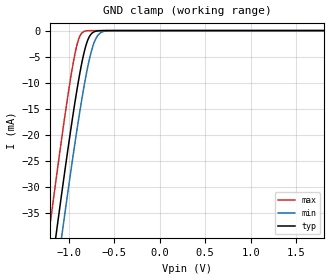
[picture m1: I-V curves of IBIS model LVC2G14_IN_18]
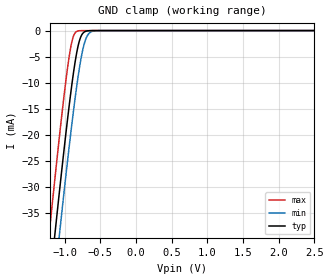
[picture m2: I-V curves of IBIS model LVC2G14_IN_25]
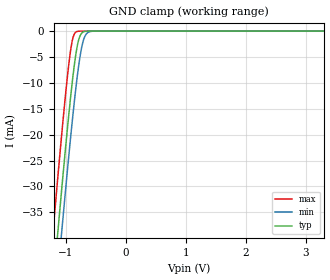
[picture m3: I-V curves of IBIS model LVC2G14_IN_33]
| TEXAS INSTRUMENTS INCORPORATED
| Standard Linear and Logic Group
| IBIS Model of SN74LVC2G14
| DUAL SCHMITT-TRIGGER INVERTER
| This file contains package information for the following:
|  SOT 6-pin (DCK) package as [Component] LVC2G14_DCK
|  SOT 6-pin (DBV) package as [Component] LVC2G14_DBV
|  NanoStar WCSP 6-pin (YEA) package as [Component] LVC2G14_YEA
|  NanoFree WCSP 6-pin (YZA) package as [Component] LVC2G14_YZA
|  NanoStar WCSP 6-pin (YEP) package as [Component] LVC2G14_YEP
|  NanoFree WCSP 6-pin (YZP) package as [Component] LVC2G14_YZP
| This device can be powered at the following Vccs:
|  1.8 volt Vcc
|  2.5 volt Vcc
|  3.3 volt Vcc
|  5 volt Vcc
| This file provides unique models under the [Model Selector] for each Vcc.
| For operation at a specific Vcc, select the appropriate model after each
| [Model Selector] keyword.
[IBIS Ver]   3.2
[Comment char]  |_char
[File Name]   sn74lvc2g14.ibs
[File Rev]   1.2 | d_die
[Date]   August 18, 2003
[Source]   Data created from TI-SPICE simulations at TI-SLL.
[Notes]   The following is an IBIS list for the LVC2G14.
   Please contact sllibis@ti.com with questions and
   comments concerning SLL IBIS models.
   -Due to the fact that the device is 5-V input/output
   tolerant, the output model has some non-monotonic
   warnings.
   -Power clamp data deleted as there is no power-clamp diode.
[Disclaimer] Property of Texas Instruments Incorporated.  Unauthorized
   reproduction and/or distribution is strictly prohibited.
   This product is protected under copyright law.
   Created  2002, (C) Copyright  2002, Texas Instruments
   Incorporated, All Rights Reserved
   UNLESS THERE IS A SIGNED, WRITTEN AGREEMENT TO THE
   CONTRARY, TEXAS INSTRUMENTS (TI) IS PROVIDING THE IBIS
   MODELS  AND WITHOUT ANY WARRANTY, EXPRESSED OR
   IMPLIED.  TI assumes no liability for:
   1) the accuracy of the IBIS models provided to your
   company;
   2) the proper functioning of these IBIS Models in your
   design or for any resulting applications; or
   3) infringement of patents, copyrights or intellectual
   property rights resulting from your use of these IBIS
   models.
   TI provides IBIS Models as a service to our customers.
   You and your company shall not distribute, sell or give
   these models to anyone else without prior written
   permission from TI.
   TI reserves the right to make changes to our products or
   to discontinue any semiconductor product or service
   without notice, and advises our customers to obtain the
   latest version of relevant information to verify, before
   placing orders, that the information being relied on is
   current.
   Please be aware that your receipt and use of the IBIS
   information provided shall serve as acceptance of these
   terms and conditions.  If you do not accept these terms,
   you should return or destroy the IBIS models and any
   other accompanying information immediately.
| Component LVC2G14_DCK 6-pin SOT
[Component]   LVC2G14_DCK
[Manufacturer]   Texas Instruments, Inc.
[Package]
|   typ   min   max
R_pkg   1.400e-02   1.100e-02   2.100e-02
L_pkg   9.480e-10   7.840e-10   1.103e-09
C_pkg   1.910e-13   1.670e-13   2.050e-13
[Pin]   signal_name   model_name   R_pin   L_pin   C_pin
1   1A   LVC2G14_IN   1.300e-02   9.840e-10   1.960e-13
2   GND   GND   2.100e-02   1.103e-09   2.050e-13
3   2A   LVC2G14_IN   1.100e-02   9.980e-10   1.970e-13
4   2Y   LVC2G14_OUT   1.300e-02   9.040e-10   1.900e-13
5   VCC   POWER   1.500e-02   7.840e-10   1.670e-13
6   1Y   LVC2G14_OUT   1.200e-02   9.160e-10   1.950e-13
| Component LVC2G14_DBV 6-pin SOT
[Component]   LVC2G14_DBV
[Manufacturer]   Texas Instruments, Inc.
[Package]
|   typ   min   max
R_pkg   2.500e-02   1.900e-02   3.700e-02
L_pkg   1.524e-09   1.260e-09   1.751e-09
C_pkg   2.450e-13   1.980e-13   2.640e-13
[Pin]   signal_name   model_name   R_pin   L_pin   C_pin
1   1A   LVC2G14_IN   2.100e-02   1.405e-09   2.460e-13
2   GND   GND   3.700e-02   1.751e-09   2.630e-13
3   2A   LVC2G14_IN   2.600e-02   1.493e-09   2.470e-13
4   2Y   LVC2G14_OUT   1.900e-02   1.620e-09   2.640e-13
5   VCC   POWER   2.400e-02   1.260e-09   1.980e-13
6   1Y   LVC2G14_OUT   2.100e-02   1.617e-09   2.500e-13
| Component LVC2G14_YEA 6-pin NanoStar WCSP
[Component]   LVC2G14_YEA
[Manufacturer]   Texas Instruments, Inc.
[Package]
|   typ   min   max
R_pkg   0.001   0.001   0.001
L_pkg   1.021nH   1.021nH   1.021nH
C_pkg   0.047pF   0.046pF   0.047pF
[Pin]   signal_name   model_name   R_pin   L_pin   C_pin
1   1A   LVC2G14_IN   0.001   0.021nH   0.046pF
2   GND   GND   0.001   0.021nH   0.047pF
3   2A   LVC2G14_IN   0.001   0.021nH   0.046pF
4   2Y   LVC2G14_OUT   0.001   0.021nH   0.046pF
5   VCC   POWER   0.001   0.021nH   0.047pF
6   1Y   LVC2G14_OUT   0.001   0.021nH   0.046pF
| Component LVC2G14_YZA 6-pin NanoFree WCSP
[Component]   LVC2G14_YZA
[Manufacturer]   Texas Instruments, Inc.
[Package]
|   typ   min   max
R_pkg   0.001   0.001   0.001
L_pkg   1.021nH   1.021nH   1.021nH
C_pkg   0.047pF   0.046pF   0.047pF
[Pin]   signal_name   model_name   R_pin   L_pin   C_pin
1   1A   LVC2G14_IN   0.001   0.021nH   0.046pF
2   GND   GND   0.001   0.021nH   0.047pF
3   2A   LVC2G14_IN   0.001   0.021nH   0.046pF
4   2Y   LVC2G14_OUT   0.001   0.021nH   0.046pF
5   VCC   POWER   0.001   0.021nH   0.047pF
6   1Y   LVC2G14_OUT   0.001   0.021nH   0.046pF
| Component LVC2G14_YEP 6-pin NanoStar WCSP
[Component]   LVC2G14_YEP
[Manufacturer]   Texas Instruments, Inc.
[Package]
|   typ   min   max
R_pkg   0.001   0.001   0.001
L_pkg   1.021nH   1.021nH   1.021nH
C_pkg   0.047pF   0.046pF   0.047pF
[Pin]   signal_name   model_name   R_pin   L_pin   C_pin
1   1A   LVC2G14_IN   0.001   0.021nH   0.046pF
2   GND   GND   0.001   0.021nH   0.047pF
3   2A   LVC2G14_IN   0.001   0.021nH   0.046pF
4   2Y   LVC2G14_OUT   0.001   0.021nH   0.046pF
5   VCC   POWER   0.001   0.021nH   0.047pF
6   1Y   LVC2G14_OUT   0.001   0.021nH   0.046pF
| Component LVC2G14_YZP 6-pin NanoFree WCSP
[Component]   LVC2G14_YZP
[Manufacturer]   Texas Instruments, Inc.
[Package]
|   typ   min   max
R_pkg   0.001   0.001   0.001
L_pkg   1.021nH   1.021nH   1.021nH
C_pkg   0.047pF   0.046pF   0.047pF
[Pin]   signal_name   model_name   R_pin   L_pin   C_pin
1   1A   LVC2G14_IN   0.001   0.021nH   0.046pF
2   GND   GND   0.001   0.021nH   0.047pF
3   2A   LVC2G14_IN   0.001   0.021nH   0.046pF
4   2Y   LVC2G14_OUT   0.001   0.021nH   0.046pF
5   VCC   POWER   0.001   0.021nH   0.047pF
6   1Y   LVC2G14_OUT   0.001   0.021nH   0.046pF
| Model LVC2G14_IN
[Model Selector]   LVC2G14_IN
LVC2G14_IN_18   1.8 volt Vcc
LVC2G14_IN_25   2.5 volt Vcc
LVC2G14_IN_33   3.3 volt Vcc
LVC2G14_IN_50   5 volt Vcc
| Model LVC2G14_OUT
[Model Selector]   LVC2G14_OUT
LVC2G14_OUT_18   1.8 volt Vcc
LVC2G14_OUT_25   2.5 volt Vcc
LVC2G14_OUT_33   3.3 volt Vcc
LVC2G14_OUT_50   5 volt Vcc
| Models and submodels in the file (8): LVC2G14_IN_18 (Input), LVC2G14_IN_25 (Input), LVC2G14_IN_33 (Input), LVC2G14_IN_50 (Input), LVC2G14_OUT_18 (Output), LVC2G14_OUT_25 (Output), LVC2G14_OUT_33 (Output), LVC2G14_OUT_50 (Output)
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[Model]   LVC2G14_IN_18
Model_type  Input
Vinl=0.7
Vinh=1.4
| variable   typ   min   max
C_comp   3.94pF   3.19pF   4.85pF
[Temperature Range]   40   100   -40
| Ambient temperature   25   85   -40
[Voltage range]   1.8   1.65   1.95
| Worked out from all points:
|   GND clamp passes 1 mA (typ) near -0.77 V on its own axis
[GND Clamp]
| LVC2G14_IN_18
|   Voltage   I(typ)   I(min)   I(max)
-5.5V     -655.2mA   -662.2mA   -646.6mA
-1.215V   -49.6mA    -57.88mA   -38.96mA
-1.135V   -39.07mA   -47.36mA   -28.42mA
-1.075V   -31.35mA   -39.6mA    -20.75mA
-1.055V   -28.82mA   -37.05mA   -18.27mA
-955mV    -16.68mA   -24.66mA   -6.874mA
-885mV    -9.098mA   -16.55mA   -1.486mA
-825mV    -3.922mA   -10.26mA   -137.1uA
-780mV    -1.472mA   -6.227mA   -17.15uA
-715mV    -205.4uA   -2.128mA   -808.5nA
-650mV    -22.01uA   -443.9uA   -37.93nA
1.8V      3.326pA    6.142pA    3.026pA
[Model]   LVC2G14_IN_25
Model_type  Input
Vinl=1.0
Vinh=1.7
| variable   typ   min   max
C_comp   4.00pF   3.04pF   5.08pF
[Temperature Range]   40   100   -40
| Ambient temperature   25   85   -40
[Voltage range]   2.5   2.3   2.7
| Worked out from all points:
|   GND clamp passes 1 mA (typ) near -0.77 V on its own axis
[GND Clamp]
| LVC2G14_IN_25
|   Voltage   I(typ)   I(min)   I(max)
-5.5V     -655.2mA   -662.2mA   -646.6mA
-1.215V   -49.6mA    -57.88mA   -38.96mA
-1.14V    -39.72mA   -48.01mA   -29.07mA
-1.12V    -37.12mA   -45.41mA   -26.48mA
-1.08V    -31.98mA   -40.25mA   -21.38mA
-1.06V    -29.44mA   -37.69mA   -18.89mA
-960mV    -17.26mA   -25.26mA   -7.377mA
-890mV    -9.597mA   -17.1mA    -1.734mA
-785mV    -1.671mA   -6.635mA   -21.67uA
-720mV    -242.5uA   -2.354mA   -1.023uA
-650mV    -22.01uA   -443.9uA   -37.93nA
2.5V      4.713pA    7.577pA    4.389pA
[Model]   LVC2G14_IN_33
Model_type  Input
Vinl=1.3
Vinh=2.2
| variable   typ   min   max
C_comp   4.01pF   3.26pF   5.21pF
[Temperature Range]   40   100   -40
| Ambient temperature   25   85   -40
[Voltage range]   3.3   3   3.6
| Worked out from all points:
|   GND clamp passes 1 mA (typ) near -0.77 V on its own axis
[GND Clamp]
| LVC2G14_IN_33
|   Voltage   I(typ)   I(min)   I(max)
-5.5V     -655.2mA   -662.2mA   -646.6mA
-1.225V   -50.93mA   -59.21mA   -40.3mA
-1.145V   -40.37mA   -48.66mA   -29.72mA
-1.12V    -37.12mA   -45.41mA   -26.48mA
-1.08V    -31.98mA   -40.25mA   -21.38mA
-1.06V    -29.44mA   -37.69mA   -18.89mA
-965mV    -17.84mA   -25.87mA   -7.89mA
-885mV    -9.098mA   -16.55mA   -1.486mA
-780mV    -1.472mA   -6.227mA   -17.15uA
-715mV    -205.4uA   -2.128mA   -808.5nA
-640mV    -15.53uA   -338.1uA   -23.69nA
3.3V      6.304pA    9.258pA    5.93pA
